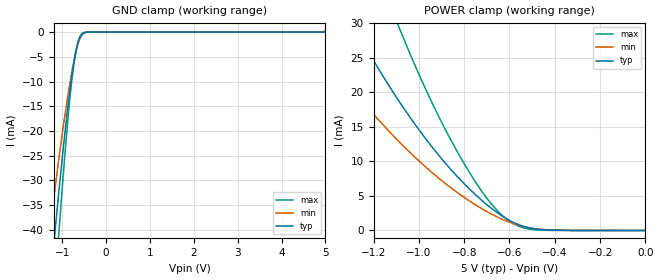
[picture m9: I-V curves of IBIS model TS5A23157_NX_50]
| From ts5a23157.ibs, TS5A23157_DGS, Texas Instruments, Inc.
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[Model]   TS5A23157_NX_50
Model_type  Terminator
| variable   typ   min   max
C_comp   5.46pF   4.93pF   5.94pF
| C_tri-state   5.46pF   4.93pF   5.94pF
[Temperature Range]   40   100   -40
| Ambient temperature   25   85   -40
[Voltage range]   5   4.5   5.5
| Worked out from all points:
|   GND clamp passes 1 mA (typ) near -0.59 V on its own axis
|   POWER clamp passes 1 mA (typ) near -0.57 V on its own axis
[GND Clamp]
| TS5A23157_NX_50
|   Voltage   I(typ)   I(min)   I(max)
-5V       -529.4mA   -428.6mA   -635.8mA
-1.28V    -51.6mA    -40.1mA    -66.49mA
-1.19V    -42.69mA   -33.43mA   -54.71mA
-1.15V    -38.86mA   -30.57mA   -49.61mA
-1.09V    -33.28mA   -26.41mA   -42.15mA
-1.07V    -31.47mA   -25.06mA   -39.71mA
-895mV    -16.83mA   -14.11mA   -19.94mA
-770mV    -8.115mA   -7.489mA   -8.825mA
-650mV    -2.367mA   -2.664mA   -2.347mA
-590mV    -955.9uA   -1.145mA   -770.1uA
-525mV    -268.1uA   -324.2uA   -148.2uA
5V        234.7pA    312.5uA    43.98pA
[POWER Clamp]
| TS5A23157_NX_50
|   Voltage   I(typ)   I(min)   I(max)
-5V       446.3mA    337.2mA    631.6mA
-1.505V   43.61mA    29.8mA     69.75mA
-1.475V   41.55mA    28.38mA    66.47mA
-1.29V    29.75mA    20.32mA    47.46mA
-1.26V    27.98mA    19.12mA    44.59mA
-1.08V    18.34mA    12.6mA     28.8mA
-965mV    13.07mA    9.044mA    20.09mA
-830mV    7.795mA    5.483mA    11.38mA
-715mV    4.147mA    3.015mA    5.326mA
-620mV    1.84mA     1.455mA    1.83mA
-505mV    325.9uA    339.7uA    158.4uA
-84.45fV  234.7pA    1.164nA    54.01pA
